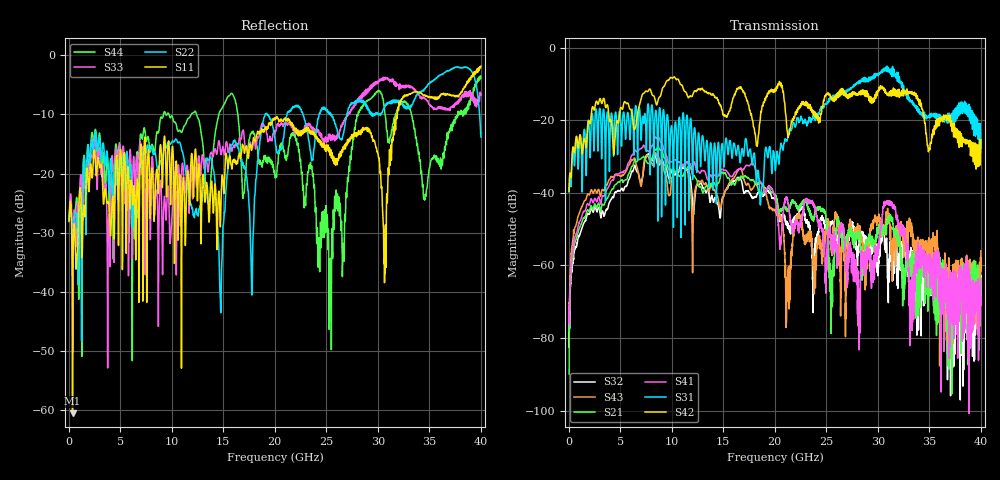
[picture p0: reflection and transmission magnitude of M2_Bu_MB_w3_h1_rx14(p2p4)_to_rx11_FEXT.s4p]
! S11 = S11
! S12 = S12
! S13 = S13
! S14 = S14
! S21 = S21
! S22 = S22
! S23 = S23
! S24 = S24
! S31 = S31
! S32 = S32
! S33 = S33
! S34 = S34
! S41 = S41
! S42 = S42
! S43 = S43
! S44 = S44
! FILE: \\englab.brocade.com\shares\Groups\SIT\Work\Shaohua\IEEE_channels\M2_Bu_MB_w3_h1_rx14(p2p4)_to_rx11_FEXT.s4p
!$DUT_CFG_DESC: Default 4-Port Configuration
!$NUMBER_PORTS: 4
!$DIFF_PORT_MAP: 1|2P|2|2P|0|UC|0|UC|
!$PORT_MAP: PNA 1|1|<<<<<<|TS 2|2|>>>>>>|PNA 2|3|<<<<<<|TS 4|4|>>>>>>|
# MHz S RI R 50.00
! FREQ  S11  S12  S13  S14
!  S21  S22  S23  S24
!  S31  S32  S33  S34
!  S41  S42  S43  S44
!  REAL  IMAG  REAL  IMAG  REAL  IMAG  REAL  IMAG
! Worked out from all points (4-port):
!   3996 points, 50 MHz to 40 GHz, reference 50 ohm
!   strongest paths, dB at 50 MHz, 10.04 GHz, 20.03 GHz, 30.02 GHz, 40 GHz:
!     S42: -39.5, -8.3, -11.8, -11.9, -25.4
!     S31: -39.7, -22.5, -33.5, -7.5, -26.8
!     S41: -75.7, -31.5, -41.4, -54.1, -70.8
!     S21: -89.9, -33.9, -40.4, -51.3, -66.5
!     S43: -72.6, -35.7, -44.8, -47.8, -56.0
!     S32: -72.4, -34.4, -41.8, -57.7, -65.5
!   lowest |S11| = -60.5 dB at 380 MHz (marker M1), VSWR 1.00, Z = 50.1 + j0.0606 ohm
!   |S11| at or under -10 dB: start of sweep to 31.89 GHz
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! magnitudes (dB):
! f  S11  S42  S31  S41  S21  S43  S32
! 50 MHz  -28.0  -39.5  -39.7  -75.7  -89.9  -72.6  -72.4
! 380 MHz  -60.5  -28.1  -28.5  -56.5  -57.8  -53.7  -59.6
! 8.58 GHz  -19.4  -15.6  -21.9  -25.0  -27.6  -29.9  -31.7
! 18.7 GHz  -12.9  -17.7  -39.6  -37.5  -40.5  -37.3  -40.2
! 21.26 GHz  -10.8  -24.3  -24.6  -42.4  -45.1  -65.4  -49.5
! 25.44 GHz  -15.9  -13.5  -14.2  -51.8  -69.6  -54.2  -47.9
! 40 GHz  -1.8  -25.4  -26.8  -70.8  -66.5  -56.0  -65.5
